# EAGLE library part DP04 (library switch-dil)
DIL/CODE SWITCH
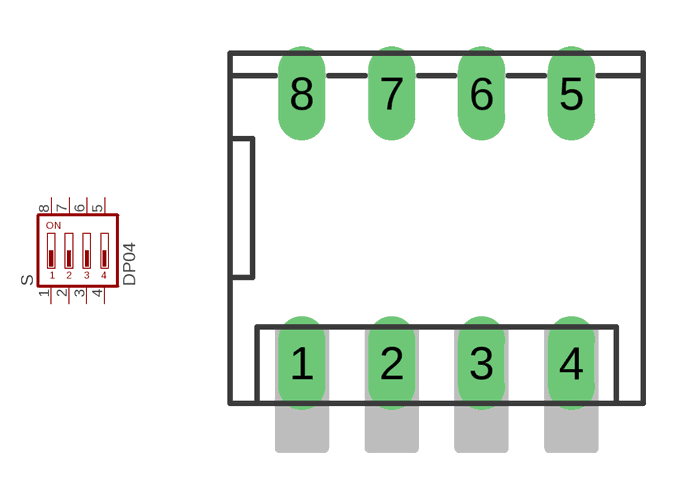
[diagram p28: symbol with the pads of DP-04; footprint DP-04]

Designator prefix S

## DP04 (MPN: DP04; OC_FARNELL: 9471600; OC_NEWARK: 73J0027)  [DP-04]
1  1  pas
2  2  pas
3  3  pas
4  4  pas
5  5  pas
6  6  pas
7  7  pas
8  8  pas

## Footprint DP-04 (pad centres in mm)
DIL/CODE SWITCH distributor Buerklin, 17G570
drill 0.813 long: 1 -3.81,-3.81; 2 -1.27,-3.81; 3 1.27,-3.81; 4 3.81,-3.81; 5 3.81,3.81; 6 1.27,3.81; 7 -1.27,3.81; 8 -3.81,3.81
